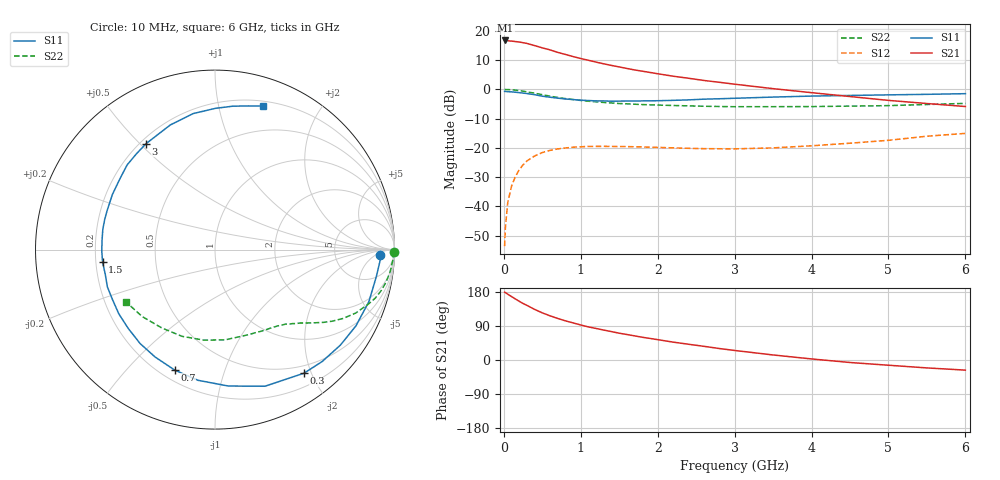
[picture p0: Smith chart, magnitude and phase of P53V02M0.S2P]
! SIEMENS Small Signal Semiconductors
! BFP183
! Si NPN RF Bipolar Junction Transistor in SOT143
! VCE = 3 V  IC = 2 mA
! Common Emitter S-Parameters:  March  1996
# GHz  S  MA  R  50
!  f  S11  S21  S12  S22
! GHz  MAG  ANG  MAG  ANG  MAG  ANG  MAG  ANG
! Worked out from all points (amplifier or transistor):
!   36 points, 10 MHz to 6 GHz, reference 50 ohm
!   highest |S21| = 16.7 dB at 20 MHz (marker M1)
!   |S21| within 3 dB of that: start of sweep to 568.2 MHz
!   unconditionally stable (mu >= 1): 2.099 GHz to 5.852 GHz
!   at 250 MHz: K = 0.12, MSG = 20.9 dB, |S12| = -25.8 dB
!   at 1.4 GHz: K = 0.67, MSG = 13.8 dB, |S12| = -19.5 dB
!   at 6 GHz: K = 0.97, MSG = 4.6 dB, |S12| = -15.0 dB
!   S11 on the Smith chart (normalised r, x): 10 MHz: 21, -9; 300 MHz: 0.38, -1.89; 700 MHz: 0.26, -0.69; 1.5 GHz: 0.23, -0.05; 3 GHz: 0.22, +0.52; 6 GHz: 0.25, +1.36
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0.01  0.9225 -2.0  6.795 178.9  0.0021 88.0  0.9991 -0.8
0.02  0.9216 -3.9  6.838 178.0  0.0043 89.1  0.9928 -1.4
0.05  0.9117 -9.3  6.769 173.7  0.0115 87.9  0.9923 -3.5
0.1  0.9052 -18.6  6.663 167.4  0.0222 78.4  0.9837 -7.2
0.2  0.8782 -37.3  6.434 155.0  0.0425 69.3  0.9542 -13.8
0.25  0.8634 -46.2  6.259 149.1  0.0513 64.4  0.9324 -16.9
0.3  0.8487 -54.2  6.084 144.2  0.0599 60.0  0.9065 -19.6
0.4  0.8106 -69.9  5.59 133.5  0.0729 52.0  0.8597 -24.3
0.5  0.7638 -84.4  5.109 124.4  0.0833 44.8  0.8108 -28.2
0.6  0.7342 -97.5  4.721 116.6  0.0908 39.2  0.7656 -31.4
0.7  0.7077 -108.5  4.281 109.7  0.0961 34.1  0.727 -33.9
0.8  0.6851 -119.2  3.948 103.4  0.0996 30.2  0.6949 -35.9
0.9  0.6693 -128.6  3.632 97.9  0.1031 26.6  0.6697 -37.6
1.1  0.6444 -146.3  3.139 87.3  0.1061 20.8  0.6269 -40.7
1.5  0.6303 -173.6  2.415 70.7  0.1054 14.0  0.5727 -46.4
1.8  0.6352 169.7  2.043 60.0  0.104 11.2  0.55 -50.6
2.2  0.649 151.7  1.678 47.2  0.1003 9.6  0.5304 -57.0
3  0.7043 123.0  1.225 25.2  0.0963 13.4  0.5053 -72.5
3.5  0.7379 109.7  1.028 13.3  0.1001 17.8  0.5059 -83.5
4.5  0.7871 89.8  0.754 -6.6  0.1203 23.8  0.517 -110.8
5.5  0.8222 76.8  0.573 -20.9  0.1584 24.1  0.5508 -137.3
6  0.8438 71.4  0.509 -26.7  0.177 20.7  0.5763 -149.8
